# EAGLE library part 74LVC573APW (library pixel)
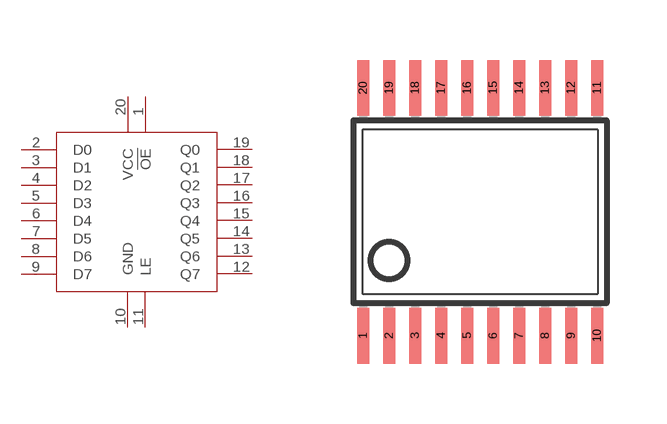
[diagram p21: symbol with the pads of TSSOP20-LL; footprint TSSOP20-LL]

Designator prefix -

## 74LVC573APW  [TSSOP20-LL]
1  !OE
2  D0
3  D1
4  D2
5  D3
6  D4
7  D5
8  D6
9  D7
10  GND
11  LE
12  Q7
13  Q6
14  Q5
15  Q4
16  Q3
17  Q2
18  Q1
19  Q0
20  VCC

## Footprint TSSOP20-LL (pad centres in mm)
Thin Shrink Small Outline Plastic 20 MAX3223-MAX3243.pdf
smd 0.3 x 1.4: 1 -2.925,-3.1; 2 -2.275,-3.1; 3 -1.625,-3.1; 4 -0.975,-3.1; 5 -0.325,-3.1; 6 0.325,-3.1; 7 0.975,-3.1; 8 1.625,-3.1; 9 2.275,-3.1; 10 2.925,-3.1; 11 2.925,3.1; 12 2.275,3.1; 13 1.625,3.1; 14 0.975,3.1; 15 0.325,3.1; 16 -0.325,3.1; 17 -0.975,3.1; 18 -1.625,3.1; 19 -2.275,3.1; 20 -2.925,3.1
